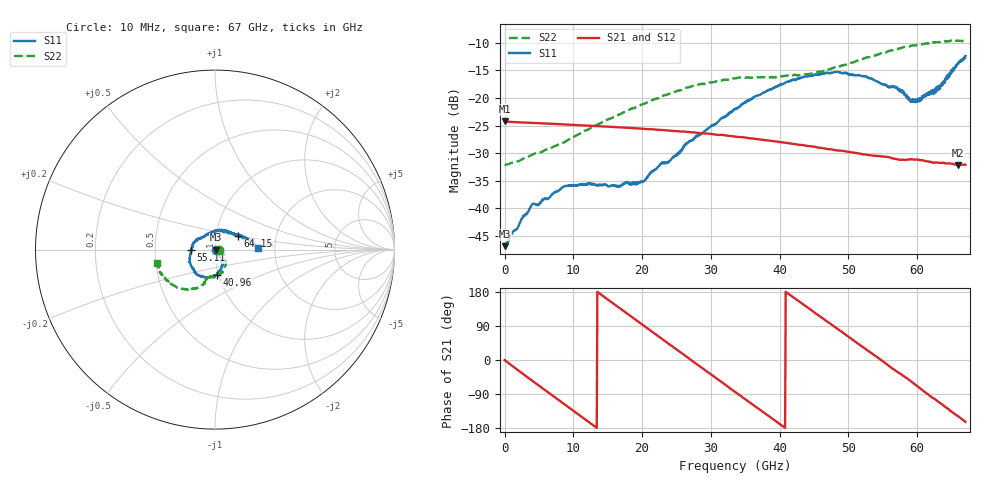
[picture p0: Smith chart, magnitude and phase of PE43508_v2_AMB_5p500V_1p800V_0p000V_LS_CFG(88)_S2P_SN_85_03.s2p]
!Keysight Technologies,N5227A,US51270237,A.10.43.00
!Date: Wednesday, August 22, 2018 17:15:50
!Correction: S11(Full 2 Port(1,3))
!S31(Full 2 Port(1,3))
!S13(Full 2 Port(1,3))
!S33(Full 2 Port(1,3))
!S2P File: Measurements: S11, S31, S13, S33:
# Hz S  dB  R 50
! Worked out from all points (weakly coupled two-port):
!   801 points, 10 MHz to 67 GHz, reference 50 ohm
!   highest |S21| = -24.26 dB at 10 MHz (marker M1); lowest = -32.2 dB at 65.91 GHz (marker M2)
!   lowest |S11| = -46.9 dB at 93.74 MHz (marker M3), VSWR 1.01, Z = 50.5 - j0.0153 ohm
!   |S11| at or under -10 dB: start of sweep to end of sweep
!   |S22| runs from -32.1 to -9.6 dB; largest |S21 - S12| = 0.00029
!   S11 on the Smith chart (normalised r, x): 10 MHz: 1.01, -0.00; 40.96 GHz: 0.98, -0.28; 55.11 GHz: 0.76, -0.00; 64.15 GHz: 1.27, +0.19; 67 GHz: 1.63, +0.03
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1e7  -46.43 -4.5  -24.26 -0.3  -24.27 -0.2  -32.09 -0.5
9.37375e7  -46.89 -1.9  -24.28 -1.4  -24.29 -1.4  -32.13 0.1
4.113138e9  -39.21 -57.1  -24.53 -55.8  -24.53 -55.8  -30.24 -3.9
8.7187e9  -36.01 -90.9  -24.79 -117.1  -24.79 -117.1  -28.02 -13.6
1.123082e10  -35.63 -96.3  -24.94 -150.3  -24.95 -150.3  -26.25 -20.7
1.935336e10  -35.26 -73.8  -25.52 102.4  -25.52 102.4  -21.49 -44.5
2.236791e10  -32.39 -61.9  -25.78 62.6  -25.77 62.5  -20.00 -53.9
2.395892e10  -31.49 -56.1  -25.92 41.6  -25.92 41.6  -19.23 -58.7
2.755964e10  -27.29 -52.5  -26.24 -5.9  -26.24 -5.9  -17.76 -70.0
3.3505e10  -22.04 -61.1  -27.00 -84.2  -27.00 -84.2  -16.43 -89.7
4.095764e10  -17.14 -86.5  -28.16 178.8  -28.15 178.8  -15.97 -102.9
4.472582e10  -15.96 -105.6  -28.78 129.8  -28.77 129.9  -15.59 -105.3
4.841028e10  -15.26 -125.5  -29.53 82.2  -29.52 82.1  -14.42 -107.3
5.510928e10  -17.49 -179.4  -30.65 -4.9  -30.63 -5.3  -11.82 -121.3
5.586291e10  -18.10 172.8  -30.74 -15.6  -30.74 -15.9  -11.48 -123.8
5.703524e10  -18.24 161.9  -31.10 -30.5  -31.09 -30.8  -11.10 -127.6
5.912868e10  -20.35 129.1  -31.09 -56.6  -31.11 -56.9  -10.52 -134.7
6.004979e10  -20.14 107.6  -31.18 -69.6  -31.19 -69.9  -10.42 -138.2
6.29806e10  -17.88 54.1  -31.71 -109.1  -31.72 -109.4  -9.90 -149.9
6.415292e10  -16.68 30.6  -31.88 -124.9  -31.94 -125.0  -9.72 -154.2
6.591141e10  -13.66 12.3  -32.16 -147.8  -32.24 -148.0  -9.60 -161.1
6.7e10  -12.39 1.8  -32.11 -163.3  -32.16 -163.3  -9.58 -166.8
